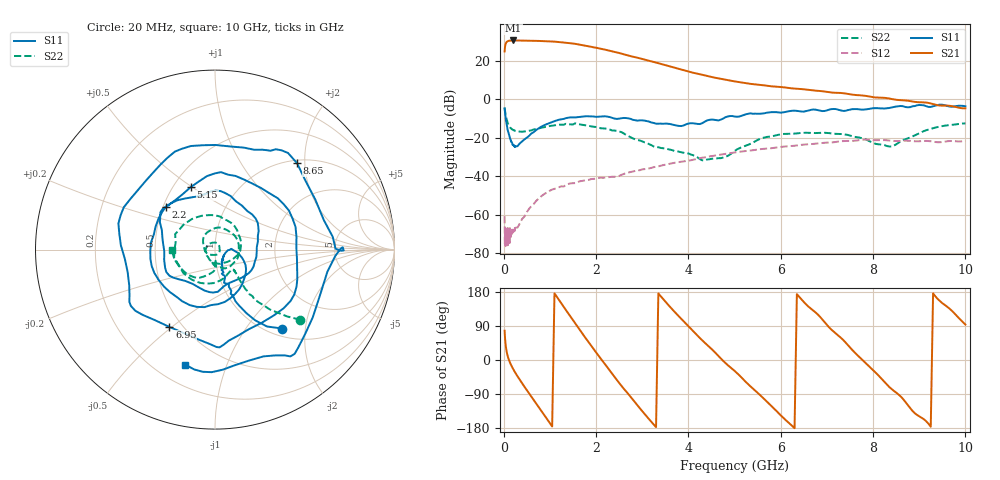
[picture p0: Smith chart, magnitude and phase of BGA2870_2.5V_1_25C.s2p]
#  HZ  S  RI  R  50.0000
! Rohde & Schwarz ZVA/B
! Temperature 25C
! Device number 1
! Measured Vcc 2.500000
! Measured Icc 0.015500
! DeltaGain  -0.112760  3dBBWHighMHz 1923.81  3dBBWLowMHz 28.34
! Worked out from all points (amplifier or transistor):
!   242 points, 20 MHz to 10 GHz, reference 50 ohm
!   highest |S21| = 30.7 dB at 210 MHz (marker M1)
!   |S21| within 3 dB of that: 30.69 MHz to 1.828 GHz (1.797 GHz wide, 193 % of centre)
!   unconditionally stable (mu >= 1): start of sweep to end of sweep
!   at 220 MHz: K = 33.58, MAG = 30.8 dB, |S12| = -67.5 dB
!   at 4 GHz: K = 3.59, MAG = 14.8 dB, |S12| = -32.0 dB
!   at 10 GHz: K = 5.62, MAG = -2.0 dB, |S12| = -21.6 dB
!   S11 on the Smith chart (normalised r, x): 20 MHz: 1.14, -1.51; 2.2 GHz: 0.52, +0.29; 5.15 GHz: 0.61, +0.50; 6.95 GHz: 0.43, -0.49; 8.65 GHz: 1.06, +1.83; 10 GHz: 0.32, -0.72
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2e7  0.375 -0.44  3.933 17.4  0.000131 0.000896  0.4754 -0.3913
4.5e7  0.1148 -0.2889  22.62 17.35  0.000418 -0.00018  0.2459 -0.2955
7.5e7  0.0502 -0.1847  31.05 8.967  0.000294 3.31e-05  0.1646 -0.2126
2.1e8  0.0434 -0.0474  31.25 -14.51  0.000109 0.000332  0.1079 -0.1163
4e8  0.0809 -0.00158  16.26 -30.09  0.000189 0.000747  0.0875 -0.1143
6e8  0.1282 -0.0184  -4.087 -33.55  0.000602 0.00154  0.0647 -0.1423
1e9  0.1514 -0.1934  -31.78 -7.616  0.00374 0.00186  -0.0818 -0.1857
1.2e9  0.0542 -0.2917  -29.16 11.72  0.00515 0.000263  -0.1765 -0.1305
1.4e9  -0.1003 -0.3193  -15.96 24.86  0.00595 -0.00193  -0.226 -0.0128
1.7e9  -0.3149 -0.1679  8.704 24.5  0.005 -0.00564  -0.151 0.1552
1.95e9  -0.3571 0.0387  20.04 10.83  0.00242 -0.00816  -0.0236 0.1924
2.2e9  -0.2729 0.2397  19.35 -4.086  -0.00102 -0.00914  0.0916 0.1479
2.65e9  0.0311 0.326  1.859 -14.36  -0.0077 -0.00924  0.1108 -0.0434
3.35e9  0.2325 -0.0094  -8.776 0.6764  -0.0174 0.00453  -0.0457 -0.0337
3.9e9  0.0497 -0.2042  -1.181 5.647  -0.008 0.0229  -0.013 0.0386
5.05e9  -0.2229 0.2744  2.391 -1.62  0.0411 -0.01  -0.0452 -0.0205
5.15e9  -0.1344 0.349  1.916 -2.002  0.0396 -0.019  -0.0564 -0.00564
6.7e9  0.0252 -0.5447  -1.128 1.299  -0.0664 0.0197  0.1323 0.0201
6.95e9  -0.2542 -0.4307  -0.2796 1.58  -0.0524 0.0526  0.1295 -0.0392
8.35e9  0.2186 0.5562  0.3435 -1.002  0.0771 -0.0354  -0.00381 -0.0592
8.65e9  0.4572 0.4813  -0.212 -0.9262  0.0525 -0.0649  0.00281 -0.0874
1e10  -0.1664 -0.6407  -0.0364 0.5848  -0.0821 0.0134  -0.2374 -0.00336
